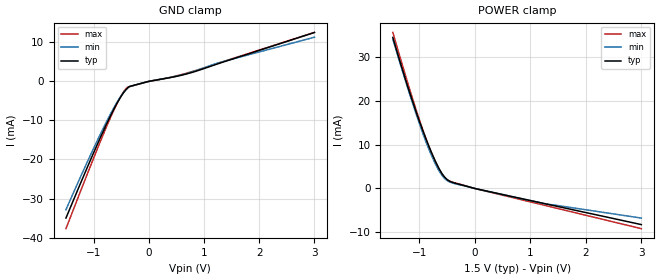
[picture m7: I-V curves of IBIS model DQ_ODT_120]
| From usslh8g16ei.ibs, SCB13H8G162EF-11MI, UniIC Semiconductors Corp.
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|   Model DQ_ODT_120
[Model] DQ_ODT_120
Model_type Input
Polarity   Non-Inverting
Enable   Active-High
Vinl =  0.615V
Vinh =  0.885V
C_comp   1.069pF   1.063pF   1.079pF
C_comp_power_clamp   0.723pF   0.708pF   0.728pF
C_comp_gnd_clamp   0.352pF   0.346pF   0.356pF
[Model Spec]
Vinh   0.885V   0.776V   0.922V
Vinl   0.615V   0.506V   0.652V
[Temperature Range]   45.000   95.000   -40.000
[Voltage Range]   1.500V   1.283V   1.575V
[C Comp Corner]
C_comp_power_clamp   0.728pF   0.723pF   0.708pF
C_comp_gnd_clamp   0.352pF   0.346pF   0.356pF
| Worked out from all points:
|   GND clamp passes 1 mA (typ) near -0.27 V on its own axis
|   POWER clamp passes 1 mA (typ) near -0.29 V on its own axis
[GND_clamp]
|Voltage   I(typ)   I(min)   I(max)
-1.5V     -35mA      -32.86mA   -37.71mA
-1.066V   -20.47mA   -19.18mA   -22.04mA
-725mV    -9.77mA    -9.216mA   -10.3mA
-508mV    -3.986mA   -3.849mA   -3.875mA
-446mV    -2.702mA   -2.657mA   -2.473mA
-384mV    -1.705mA   -1.72mA    -1.486mA
-353mV    -1.333mA   -1.364mA   -1.366mA
-12mV     -45.18uA   -45.22uA   -46.42uA
391mV     980.9uA    1.014mA    1.029mA
794mV     2.339mA    2.473mA    2.547mA
1.29V     4.679mA    4.861mA    4.802mA
3V        12.51mA    11.31mA    12.54mA
[POWER_clamp]
|Voltage   I(typ)   I(min)   I(max)
-1.476V   34.46mA    34.07mA    35.6mA
-1.166V   21.61mA    21.25mA    22.36mA
-1.011V   15.83mA    15.29mA    16.17mA
-887mV    11.58mA    10.92mA    11.62mA
-763mV    7.726mA    7.071mA    7.614mA
-670mV    5.185mA    4.631mA    5.078mA
-577mV    3.151mA    2.773mA    3.063mA
-515mV    2.225mA    1.97mA     2.165mA
-391mV    1.354mA    1.21mA     1.409mA
12mV      -32.92uA   -33.14uA   -36.64uA
1.283V    -3.52mA    -3.543mA   -3.918mA
3V        -8.23mA    -6.747mA   -9.16mA
